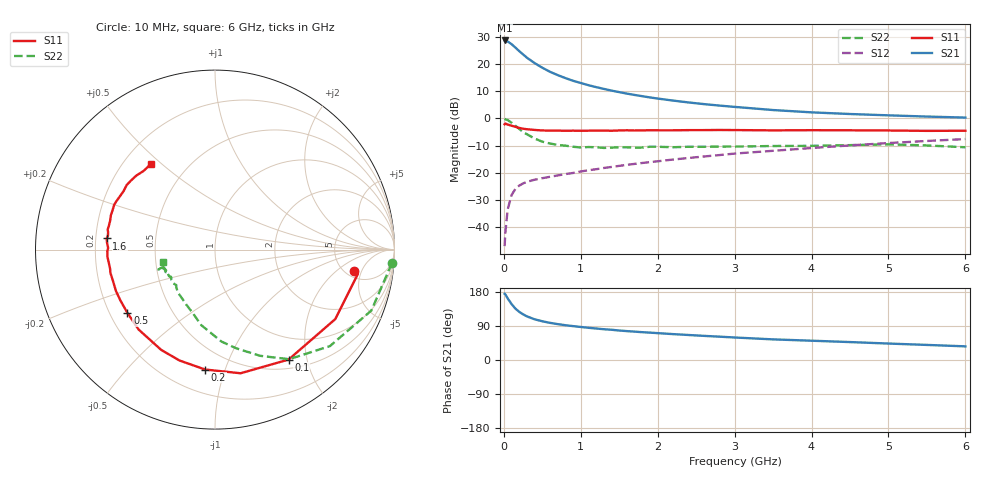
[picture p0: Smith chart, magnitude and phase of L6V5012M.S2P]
!  INFINEON TECHNOLOGIES Small Signal Semiconductors
! BFR380L3 , Si-NPN RF-Transistor in TSLP-3-1
!  Vce=0.5 V,  Ic=12.5 mA
! Common Emitter S-Parameters:  07. March 2005
#  GHz  S  MA  R  50
! f  S11  S21  S12  S22
! GHz  Mag  Ang  Mag  Ang  Mag  Ang  Mag  Ang
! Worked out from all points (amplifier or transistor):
!   36 points, 10 MHz to 6 GHz, reference 50 ohm
!   highest |S21| = 28.7 dB at 10 MHz (marker M1)
!   |S21| within 3 dB of that: start of sweep to 165.2 MHz
!   unconditionally stable (mu >= 1): 1.711 GHz to 5.945 GHz
!   at 250 MHz: K = 0.32, MSG = 23.7 dB, |S12| = -23.9 dB
!   at 1.4 GHz: K = 0.95, MSG = 14.0 dB, |S12| = -17.8 dB
!   at 6 GHz: K = 1.00, MSG = 3.9 dB, |S12| = -7.6 dB
!   S11 on the Smith chart (normalised r, x): 10 MHz: 5.97, -3.60; 100 MHz: 0.63, -1.69; 200 MHz: 0.35, -0.86; 500 MHz: 0.27, -0.30; 1.6 GHz: 0.25, +0.05; 6 GHz: 0.31, +0.46
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0.01  0.7822 -8.6  27.16 174.7  0.0045 84.7  0.9881 -4.4
0.02  0.8078 -9.6  26.97 173.2  0.0081 85.7  0.9654 -8.9
0.05  0.7739 -30.0  25.98 162.5  0.0213 76.3  0.935 -21.3
0.1  0.7373 -56.2  23.23 147.7  0.039 64.2  0.8362 -40.0
0.15  0.7036 -78.3  20.14 135.8  0.0508 55.9  0.7374 -55.9
0.2  0.6704 -94.7  17.3 127.0  0.0584 50.7  0.6435 -66.9
0.25  0.6488 -107.7  15.03 120.5  0.064 46.5  0.563 -77.8
0.3  0.6342 -118.2  13.1 115.1  0.0686 45.1  0.5134 -86.0
0.4  0.6159 -133.7  10.41 107.4  0.0749 42.8  0.4278 -100.3
0.5  0.6022 -144.1  8.57 102.2  0.0799 42.9  0.3752 -109.2
0.6  0.5984 -151.8  7.212 98.0  0.0848 43.6  0.3467 -117.2
0.7  0.5981 -157.3  6.269 94.7  0.0898 44.9  0.3272 -124.4
0.8  0.5946 -162.8  5.528 91.8  0.095 45.9  0.3168 -130.5
0.9  0.597 -167.4  4.93 89.4  0.0997 47.5  0.3022 -135.5
1.1  0.5967 -173.3  4.09 85.0  0.1118 49.6  0.2985 -141.0
1.3  0.6001 -179.1  3.499 81.2  0.1231 51.5  0.2876 -148.3
1.6  0.6068 174.1  2.866 76.2  0.1405 53.6  0.2954 -153.9
2.2  0.606 164.5  2.133 68.3  0.176 56.3  0.2959 -156.8
3.5  0.6046 147.5  1.429 54.4  0.2548 57.0  0.3119 -161.0
4.5  0.6063 140.9  1.208 47.3  0.32 56.1  0.3238 -161.0
5.5  0.5919 132.2  1.084 39.8  0.3862 52.6  0.3195 -162.5
6  0.5955 127.0  1.039 36.0  0.4188 50.5  0.2955 -167.0
